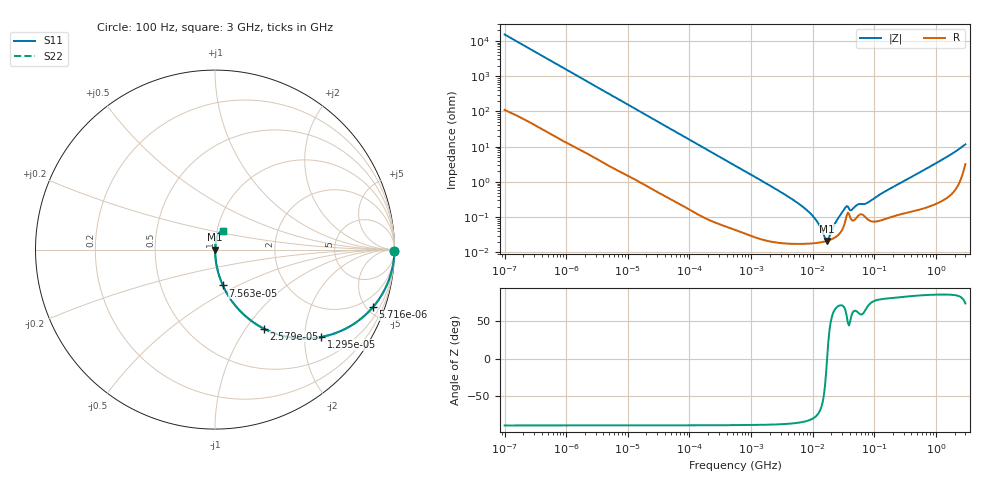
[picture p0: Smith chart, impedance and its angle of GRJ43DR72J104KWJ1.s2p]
!Murata Part Number: GRJ43DR72J104KWJ1
!These Parameters are Measured in Series Mode Connection
!Data Generated on Jun 19, 2026
!  o--ll--o
!Port1  Port2
!  o------o
!Operation Temp=25[degC], DC Bias Voltage=0[V]
!Freq. Start=100[Hz] Stop=3[GHz] 401[Steps]
# Hz S RI R 50
!Freq.(Hz) S11(Real) S11(Imag) S21(Real) S21(Imag) S12(Real) S12(Imag) S22(Real) S22(Imag)
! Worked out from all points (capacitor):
!   401 points, 100 Hz to 3 GHz, reference 50 ohm
!   read as one part in series: C = 104 nF near 109 Hz
!   lowest |Z| = 21.3 mohm at 17.14 MHz (marker M1)
!   series resonance near 17.09 MHz, so ESL is about 830 pH
!   S11 on the Smith chart (normalised r, x): 100 Hz: open; 5.716 kHz: 1.05, -5.45; 12.95 kHz: 1.02, -2.42; 25.79 kHz: 1.01, -1.22; 75.63 kHz: 1.00, -0.42; 3 GHz: 1.06, +0.22
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100  0.9999 -0.00657  9.07e-05 0.00657  9.07e-05 0.00657  0.9999 -0.00657
1788  0.9858 -0.1138  0.0142 0.1138  0.0142 0.1138  0.9858 -0.1138
5716  0.879 -0.3216  0.121 0.3216  0.121 0.3216  0.879 -0.3216
12951  0.5927 -0.4865  0.4073 0.4865  0.4073 0.4865  0.5927 -0.4865
25785  0.2729 -0.4406  0.7271 0.4406  0.7271 0.4406  0.2729 -0.4406
31977  0.1974 -0.3931  0.8026 0.3931  0.8026 0.3931  0.1974 -0.3931
75630  0.0439 -0.1996  0.9561 0.1996  0.9561 0.1996  0.0439 -0.1996
178874  0.00876 -0.088  0.9912 0.088  0.9912 0.088  0.00876 -0.088
547723  0.00129 -0.0292  0.9987 0.0292  0.9987 0.0292  0.00129 -0.0292
4323298  0.000189 -0.0035  0.9998 0.0035  0.9998 0.0035  0.000189 -0.0035
9794414  0.000182 -0.00112  0.9998 0.00112  0.9998 0.00112  0.000182 -0.00112
1.268047e7  0.00019 -0.000581  0.9998 0.000581  0.9998 0.000581  0.00019 -0.000581
1.572531e7  0.000205 -0.000161  0.9998 0.000161  0.9998 0.000161  0.000205 -0.000161
1.713898e7  0.000213 5.9e-06  0.9998 -5.9e-06  0.9998 -5.9e-06  0.000213 5.9e-06
1.867972e7  0.000224 0.000175  0.9998 -0.000175  0.9998 -0.000175  0.000224 0.000175
2.418395e7  0.000283 0.000722  0.9997 -0.000722  0.9997 -0.000722  0.000283 0.000722
3.412477e7  0.00083 0.00172  0.9992 -0.00172  0.9992 -0.00172  0.00083 0.00172
4.231884e7  0.000855 0.00133  0.9991 -0.00133  0.9991 -0.00133  0.000855 0.00133
5.478864e7  0.0011 0.00204  0.9989 -0.00204  0.9989 -0.00204  0.0011 0.00204
7.405258e7  0.000946 0.00227  0.9991 -0.00227  0.9991 -0.00227  0.000946 0.00227
1.751444e8  0.00101 0.00622  0.999 -0.00622  0.999 -0.00622  0.00101 0.00622
3e9  0.0423 0.1041  0.9577 -0.1041  0.9577 -0.1041  0.0423 0.1041
